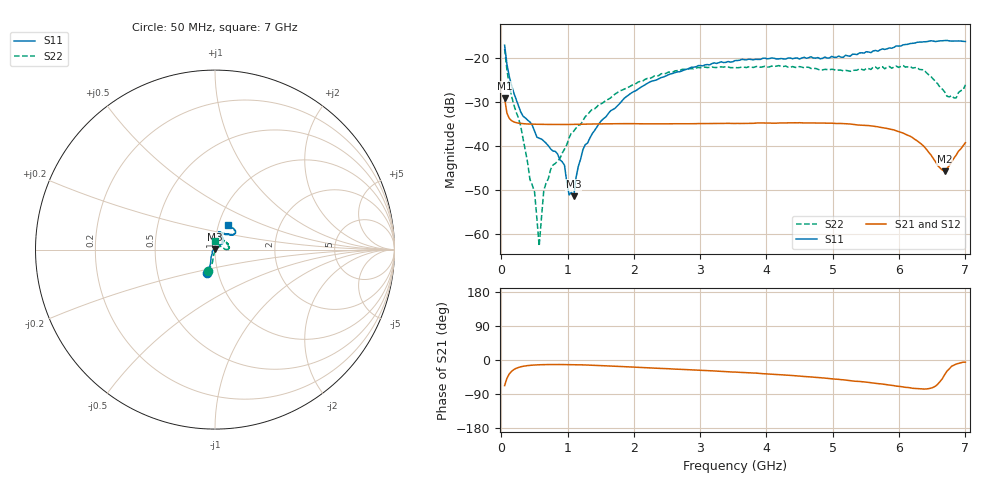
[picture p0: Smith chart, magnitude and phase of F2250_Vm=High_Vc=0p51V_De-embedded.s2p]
! Integrated Device Technology
! Corporate Headquarters
! 6024 Silver Creek Valley Road
! San Jose, CA 95138  USA
! Phone:  1-408-284-8200
! Toll Free:  1-800-223-1366
! Webpage:  http://www.idt.com/
! Timing and RF Division
! 515 Groton Road, Suite 102
! Westford, MA 01886-6024
! Device:  F2250
! Description: Voltage Variable RF Attenuator
! Frequency:  50.0 -  6000.00 MHz
! Package:  3x3 mm Thin QFN Plastic Package: 16 pin
! Ports:  2 RF, 3 DC
!  Pin  1  = GND
!  Pin  2  = NC
!  Pin  3  = RF1  = Port 1
!  Pin  4  = NC
!  Pin  5  = GND
!  Pin  6  = GND
!  Pin  7  = GND
!  Pin  8  = GND
!  Pin  9  = NC
!  Pin 10  = RF2  = Port 2
!  Pin 11  = NC
!  Pin 12  = GND
!  Pin 13  = GND
!  Pin 14  = VCNTRL
!  Pin 15  = VDD
!  Pin 16  = VMODE
! Vcntrl:  0.510 Volts
! Vmode:  +3.300 Volts
! Vdd:  +3.30  Volts
! Current:  1.268 mA
! Data:  The device was measured on a the F2250 evaluation board which has
!  individual transmission lines to the RF pins.  Data was collected
!  using a calibrated network analyzer.  The evaluation board was
!  de-embedded using a TRL calibration technique.
!  The reference plane is the edge of the package pin.
! Misc:  SN 10
!  Action Tracker AT0258
! Date Measured:  2014-11-26
! Date:  2015-10-15  MJV
! Note:
!  Integrated Device Technology supplies this data as a sample of measured
!  data at the package pin for this product.  Your particular data for this
!  product may vary.
!  Data was taken at 25 degrees C.
!  Integrated Device Technology reserves the right to change this data at anytime.
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# GHz S dB R 50
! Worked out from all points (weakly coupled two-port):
!   201 points, 50 MHz to 7 GHz, reference 50 ohm
!   highest |S21| = -29.21 dB at 50 MHz (marker M1); lowest = -45.7 dB at 6.687 GHz (marker M2)
!   lowest |S11| = -51.4 dB at 1.093 GHz (marker M3), VSWR 1.01, Z = 50 + j0.269 ohm
!   |S11| at or under -10 dB: start of sweep to end of sweep
!   |S22| runs from -62.7 to -18.0 dB; largest |S21 - S12| = 4.8e-05
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0.05  -17.17 -108.5  -29.21 -67.6  -29.21 -67.6  -18.00 -107.3
0.08475  -21.46 -107.4  -32.53 -48.4  -32.53 -48.4  -22.73 -101.1
0.189  -28.00 -119.8  -34.53 -25.3  -34.53 -25.3  -30.67 -103.9
0.29325  -32.28 -127.2  -34.88 -18.0  -34.88 -18.0  -35.50 -98.0
0.43225  -34.57 -145.1  -35.03 -14.1  -35.03 -14.1  -47.57 -101.8
0.50175  -36.64 -147.5  -35.06 -13.2  -35.06 -13.2  -50.42 -100.9
0.57125  -38.24 -161.1  -35.09 -12.6  -35.09 -12.6  -62.67 -54.2
0.64075  -38.86 -162.4  -35.11 -12.2  -35.11 -12.2  -50.08 32.8
0.745  -40.67 -173.6  -35.12 -12.0  -35.12 -12.0  -45.28 44.8
0.9535  -44.36 170.9  -35.12 -12.0  -35.13 -12.0  -40.70 50.0
1.023  -51.06 139.8  -35.12 -12.2  -35.12 -12.2  -38.15 43.7
1.0925  -51.39 88.7  -35.10 -12.4  -35.10 -12.3  -36.65 43.0
1.2315  -40.80 40.1  -35.06 -12.9  -35.06 -12.9  -34.27 33.3
1.6485  -32.02 40.9  -34.99 -15.8  -34.99 -15.8  -29.11 37.4
2.37825  -24.75 46.6  -34.96 -21.9  -34.96 -21.9  -24.02 41.7
3.525  -20.66 71.7  -34.90 -31.8  -34.90 -31.9  -22.22 66.2
4.7065  -20.06 71.9  -34.76 -45.3  -34.76 -45.3  -22.47 66.3
5.85325  -17.79 40.5  -36.14 -66.0  -36.15 -66.2  -21.98 16.9
6.3745  -16.41 40.9  -40.07 -76.6  -40.08 -76.7  -22.75 0.5
6.68725  -16.12 47.8  -45.73 -38.8  -45.71 -38.5  -27.77 22.6
6.861  -16.22 54.5  -42.06 -10.7  -42.03 -10.7  -29.11 58.8
7  -16.33 62.4  -39.25 -5.6  -39.22 -5.8  -26.13 89.3
